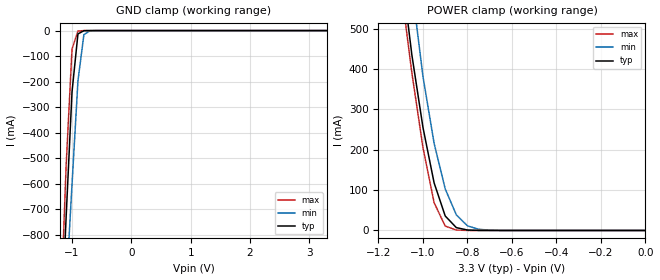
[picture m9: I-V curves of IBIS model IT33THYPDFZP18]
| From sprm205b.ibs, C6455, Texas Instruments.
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|   Model IT33THYPDFZP18
[Model]   IT33THYPDFZP18
Model_type   Input
Polarity   Non-Inverting
Vinl =   0.8000V
Vinh =   2.0000V
C_comp   0.4970pF   0.4510pF   0.5460pF
[Temperature Range]   25.0000   0.1250k   -40.0000
[Pullup Reference]   3.3000V   3.0000V   3.6000V
[Pulldown Reference]   0.000V   0.000V   0.000V
[POWER Clamp Reference]   3.3000V   3.0000V   3.6000V
[GND Clamp Reference]   0.000V   0.000V   0.000V
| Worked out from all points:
|   GND clamp passes 1 mA (typ) near -0.80 V on its own axis
|   POWER clamp passes 1 mA (typ) near -0.79 V on its own axis
[GND_clamp]
| voltage   I(typ)   I(min)   I(max)
-3.3V     -15.87A    -14.33A    -17.08A
-1.2V     -1.259A    -1.45A     -1.156A
-1.1V     -733.9mA   -1.018A    -533.6mA
-1V       -239.9mA   -601.9mA   -72.24mA
-900mV    -13.15mA   -197.2mA   -1.655mA
-800mV    -419.7uA   -16.01mA   -63.3uA
-700mV    -31uA      -1.111mA   -30.04uA
3.3V      95.11nA    98.08nA    329.9nA
[POWER_clamp]
| voltage   I(typ)   I(min)   I(max)
-3.3V     13.82A     12.46A     14.94A
-1.1V     659.5mA    849.4mA    605mA
-1.05V    434.5mA    602.9mA    390.3mA
-1V       254.9mA    380.7mA    204.9mA
-950mV    117.9mA    215.7mA    68.66mA
-900mV    35.85mA    102.9mA    10.85mA
-850mV    7.018mA    38.47mA    1.067mA
-800mV    1.123mA    11.47mA    96.7uA
-750mV    171.4uA    3.055mA    9.144uA
-700mV    26.15uA    783uA      1.258uA
0V        95.11nA    65.53nA    353.6nA
